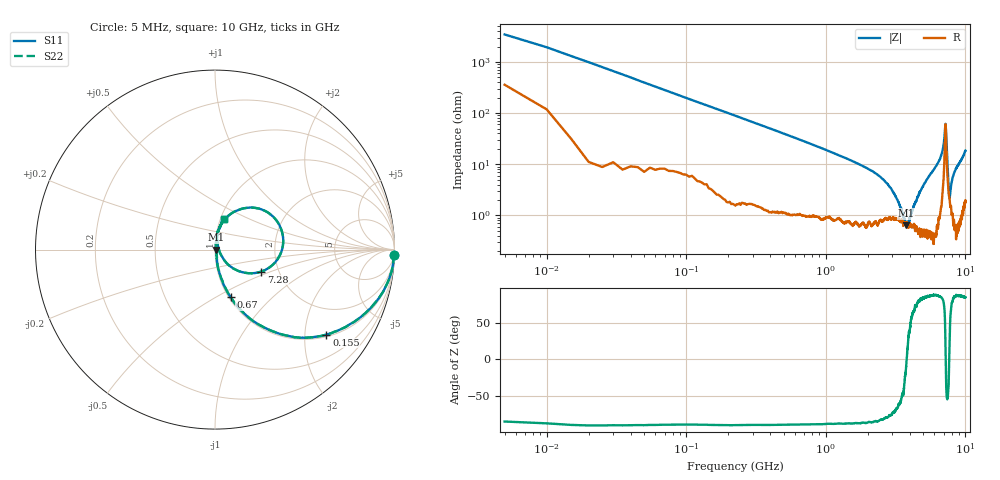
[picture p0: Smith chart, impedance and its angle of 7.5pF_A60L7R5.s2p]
! Amotech Co.,Ltd.
! http://www.amotech.co.kr/
! Part Number: A60L7R5
! These Parameters are Measured in Series Mode Connection
! Operation Temp=25[degC], DC Bias Voltage=0[V]
! Freq. Start=5[MHz] Stop=10[GHz], 2000[Steps]
! Date: Monday, July 14, 2020, 09:53:06
# GHZ S RI R 50.000000
!Freq.(Hz) S11(Real) S11(Imag) S21(Real) S21(Imag) S12(Real) S12(Imag) S22(Real) S22(Imag)
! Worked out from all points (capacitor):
!   2000 points, 5 MHz to 10 GHz, reference 50 ohm
!   read as one part in series: C = 8.03 pF near 55 MHz
!   lowest |Z| = 644 mohm at 3.76 GHz (marker M1)
!   series resonance near 3.794 GHz, so ESL is about 220 pH
!   S11 on the Smith chart (normalised r, x): 5 MHz: 8, -69; 155 MHz: 1.06, -2.57; 670 MHz: 1.02, -0.59; 7.28 GHz: 1.63, -0.43; 10 GHz: 1.04, +0.37
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0.005  0.9962 -0.0286  0.00382 0.0286  0.00382 0.0286  0.9962 -0.0286
0.075  0.8675 -0.3253  0.1325 0.3253  0.1325 0.3253  0.8675 -0.3253
0.155  0.6206 -0.4736  0.3794 0.4736  0.3794 0.4736  0.6206 -0.4736
0.355  0.2458 -0.4187  0.7542 0.4187  0.7542 0.4187  0.2458 -0.4187
0.67  0.0869 -0.2652  0.9131 0.2652  0.9131 0.2652  0.0869 -0.2652
1.675  0.0176 -0.1016  0.9824 0.1016  0.9824 0.1016  0.0176 -0.1016
2.62  0.0104 -0.0466  0.9896 0.0466  0.9896 0.0466  0.0104 -0.0466
3.34  0.00888 -0.0147  0.9911 0.0147  0.9911 0.0147  0.00888 -0.0147
3.76  0.0063 -0.00112  0.9937 0.00112  0.9937 0.00112  0.0063 -0.00112
3.915  0.00594 0.00349  0.9941 -0.00349  0.9941 -0.00349  0.00594 0.00349
4.285  0.00673 0.0138  0.9933 -0.0138  0.9933 -0.0138  0.00673 0.0138
5.005  0.00608 0.0379  0.9939 -0.0379  0.9939 -0.0379  0.00608 0.0379
6.67  0.0322 0.1343  0.9678 -0.1343  0.9678 -0.1343  0.0322 0.1343
6.955  0.0826 0.1954  0.9174 -0.1954  0.9174 -0.1954  0.0826 0.1954
7.105  0.2204 0.2329  0.7796 -0.2329  0.7796 -0.2329  0.2204 0.2329
7.2  0.3788 0.0726  0.6212 -0.0726  0.6212 -0.0726  0.3788 0.0726
7.28  0.2584 -0.1225  0.7416 0.1225  0.7416 0.1225  0.2584 -0.1225
7.415  0.0738 -0.0841  0.9262 0.0841  0.9262 0.0841  0.0738 -0.0841
7.605  0.0257 -0.0131  0.9743 0.0131  0.9743 0.0131  0.0257 -0.0131
7.675  0.0217 0.00272  0.9783 -0.00272  0.9783 -0.00272  0.0217 0.00272
8.335  0.0107 0.0688  0.9893 -0.0688  0.9893 -0.0688  0.0107 0.0688
10  0.0502 0.1722  0.9498 -0.1722  0.9498 -0.1722  0.0502 0.1722
